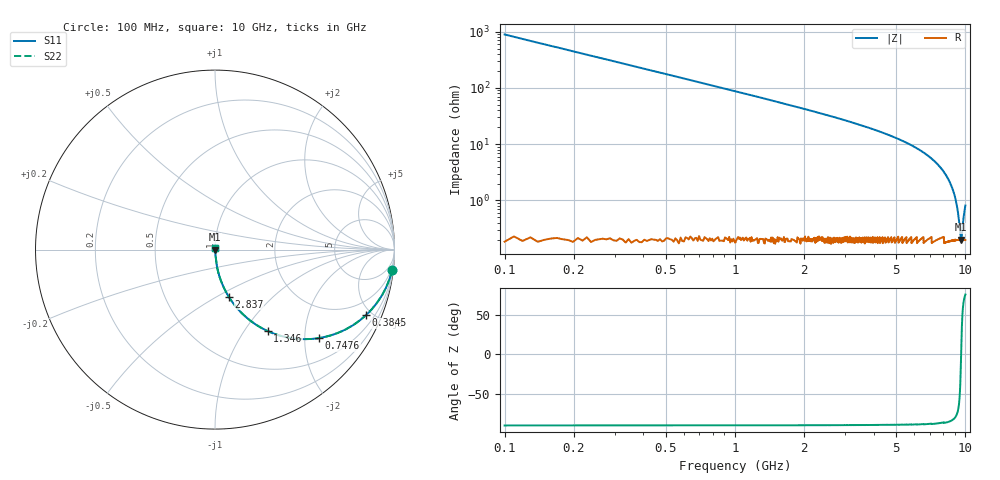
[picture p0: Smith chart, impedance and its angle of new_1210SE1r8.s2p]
!	AVX	Thin	Film	Operation	Date:	April 2007
!	Description:	Accu-P®	"Series,"	Thin	"Film,"	"SMD,"	RF	Capacitor
!	Part	Number:	12101J1R8ABT
!	100	MHz	-	6.05	GHz
!	Serial	Measurements
#	MHZ	S	MA	R	50
!	S11	S21	S12	S22
!	dB	Phase	dB	Phase	dB	Phase	dB	Phase
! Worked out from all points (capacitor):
!   1010 points, 100 MHz to 10 GHz, reference 50 ohm
!   read as one part in series: C = 1.8 pF near 149.1 MHz
!   lowest |Z| = 200 mohm at 9.578 GHz (marker M1)
!   series resonance near 9.581 GHz, so ESL is about 150 pH
!   S11 on the Smith chart (normalised r, x): 100 MHz: 1, -18; 384.5 MHz: 1.00, -4.59; 747.6 MHz: 1.00, -2.35; 1.346 GHz: 1.00, -1.29; 2.837 GHz: 1.00, -0.57; 10 GHz: 1.00, +0.02
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100  0.994 -6.5  0.112 83.5  0.112 83.5  0.994 -6.5
237.364  0.966 -15.0  0.259 74.9  0.259 74.9  0.966 -15.0
384.539  0.917 -23.5  0.399 66.4  0.399 66.4  0.917 -23.5
551.338  0.847 -32.0  0.53 57.9  0.53 57.9  0.847 -32.0
747.572  0.761 -40.3  0.647 49.6  0.647 49.6  0.761 -40.3
1032.111  0.645 -49.7  0.762 40.2  0.762 40.2  0.645 -49.7
1346.085  0.541 -57.1  0.84 32.7  0.84 32.7  0.541 -57.1
1758.176  0.436 -63.9  0.898 25.9  0.898 25.9  0.436 -63.9
2837.463  0.273 -73.8  0.96 15.8  0.96 15.8  0.273 -73.8
3406.541  0.221 -76.7  0.973 12.8  0.973 12.8  0.221 -76.7
5054.906  0.125 -81.9  0.99 7.2  0.99 7.2  0.125 -81.9
6703.271  0.067 -84.5  0.996 3.8  0.996 3.8  0.067 -84.5
7733.499  0.04 -84.8  0.997 2.3  0.997 2.3  0.04 -84.8
8351.635  0.025 -84.0  0.998 1.5  0.998 1.5  0.025 -84.0
8812.785  0.016 -81.7  0.998 0.9  0.998 0.9  0.016 -81.7
9087.512  0.00995 -77.9  0.998 0.6  0.998 0.6  0.00995 -77.9
9303.37  0.00577 -69.5  0.998 0.3  0.998 0.3  0.00577 -69.5
9519.227  0.00233 -30.8  0.998 0.1  0.998 0.1  0.00233 -30.8
9578.097  0.002 -1.6  0.998 0.0  0.998 0.0  0.002 -1.6
9636.967  0.00227 28.2  0.998 -0.1  0.998 -0.1  0.00227 28.2
9852.825  0.00553 68.5  0.998 -0.3  0.998 -0.3  0.00553 68.5
10000  0.00814 75.3  0.998 -0.5  0.998 -0.5  0.00814 75.3
